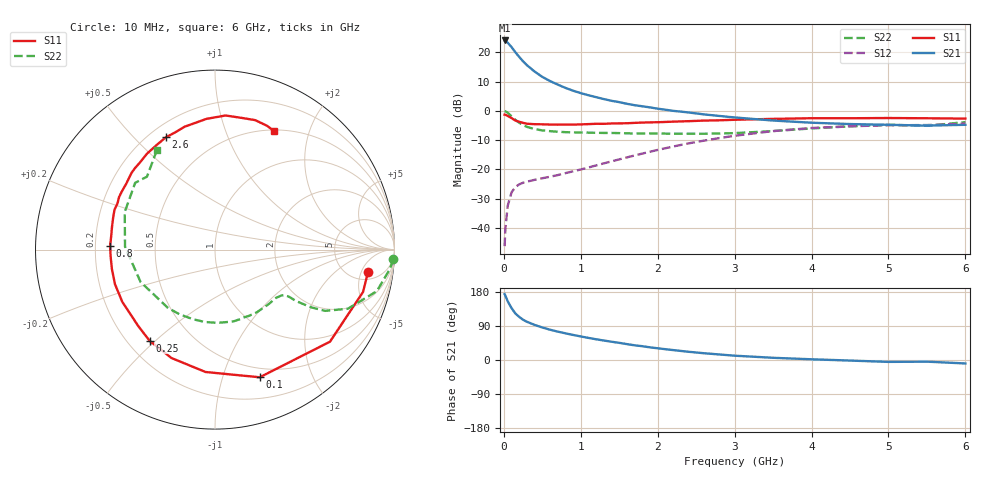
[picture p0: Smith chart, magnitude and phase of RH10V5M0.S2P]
! SIEMENS Small Signal Semiconductors
! BFR106
! Si NPN RF Bipolar Junction Transistor in SOT23
! VCE = 10 V  IC = 5 mA
! Common Emitter S-Parameters:  August  1996
# GHz  S  MA  R  50
!  f  S11  S21  S12  S22
! GHz  MAG  ANG  MAG  ANG  MAG  ANG  MAG  ANG
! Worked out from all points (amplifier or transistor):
!   36 points, 10 MHz to 6 GHz, reference 50 ohm
!   highest |S21| = 24.0 dB at 10 MHz (marker M1)
!   |S21| within 3 dB of that: start of sweep to 121 MHz
!   unconditionally stable (mu >= 1): 633.4 MHz to 1.849 GHz; 5.035 GHz to end of sweep
!   at 250 MHz: K = 0.50, MSG = 20.7 dB, |S12| = -24.5 dB
!   at 1.4 GHz: K = 1.13, MAG = 8.2 dB, |S12| = -17.2 dB
!   at 6 GHz: K = 1.02, MAG = -1.1 dB, |S12| = -4.3 dB
!   S11 on the Smith chart (normalised r, x): 10 MHz: 7.01, -6.70; 100 MHz: 0.40, -1.33; 250 MHz: 0.29, -0.48; 800 MHz: 0.26, +0.02; 2.6 GHz: 0.27, +0.62; 6 GHz: 0.52, +1.49
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0.01  0.8619 -8.2  15.94 174.0  0.0049 88.5  0.9933 -3.1
0.02  0.8579 -16.0  15.79 169.7  0.0097 83.4  0.9815 -6.2
0.05  0.8207 -38.7  14.59 155.1  0.0239 69.7  0.9309 -14.4
0.1  0.7537 -70.7  12.29 137.0  0.0406 56.4  0.8104 -24.0
0.15  0.684 -94.4  10.03 122.7  0.0501 48.0  0.7016 -29.1
0.2  0.6509 -111.9  8.332 113.7  0.0556 43.6  0.6275 -30.9
0.25  0.625 -125.7  7.021 106.2  0.0594 40.9  0.5706 -31.8
0.3  0.6034 -135.2  6.031 100.9  0.0618 40.4  0.5341 -32.4
0.4  0.5929 -150.6  4.692 92.6  0.0665 40.9  0.4885 -32.5
0.5  0.5896 -161.0  3.807 85.8  0.0708 43.1  0.4646 -33.1
0.6  0.5845 -169.5  3.234 80.0  0.0751 45.9  0.4509 -34.5
0.8  0.5846 178.0  2.472 70.5  0.0865 51.7  0.4333 -38.5
0.9  0.5831 172.9  2.212 66.1  0.0928 54.6  0.4299 -40.6
1.1  0.5947 162.6  1.85 58.3  0.108 59.5  0.4254 -46.4
1.6  0.615 143.9  1.321 41.9  0.1606 65.7  0.4144 -63.1
2.2  0.6552 125.3  1.003 26.2  0.2463 63.8  0.4085 -88.0
2.6  0.6829 113.6  0.872 17.9  0.3102 58.9  0.4067 -107.7
3.5  0.73 93.7  0.684 5.8  0.4522 42.6  0.4522 -156.5
4.5  0.7487 78.5  0.596 -1.5  0.5461 22.1  0.5447 157.4
5  0.7553 72.7  0.579 -5.0  0.5687 13.5  0.5799 140.1
5.5  0.7481 67.2  0.56 -4.4  0.5728 8.9  0.5557 133.0
6  0.738 63.4  0.579 -9.1  0.6081 0.7  0.6433 120.1
